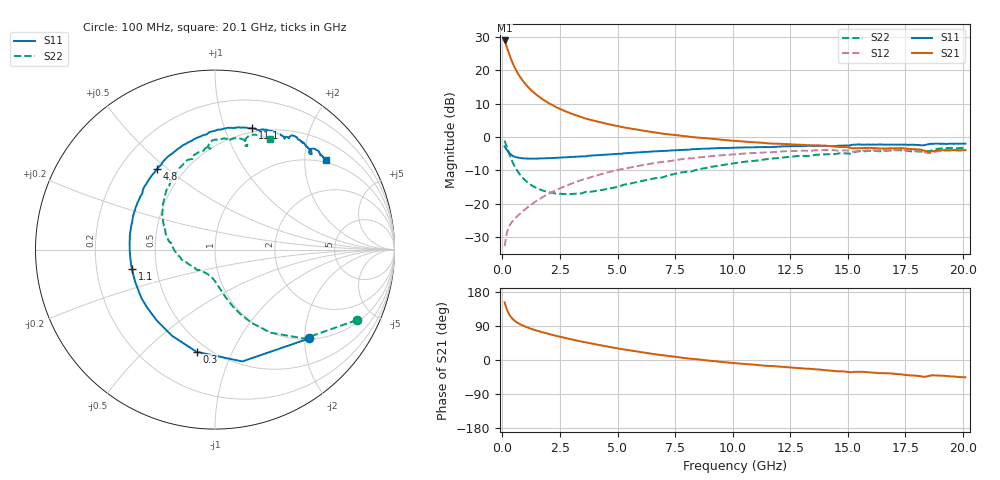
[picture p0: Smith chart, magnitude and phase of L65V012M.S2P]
!  Infineon Technologies AG
! BFR380L3 , PF131585-7, No.6, Th 09.10.01, soldered on pcb-board, measured with PP GSG850
!  Vce=5.0 V,  Ic=12.5 mA
! Common Emitter S-Parameters:  15. November 2001
#  GHz  S  MA  R  50
! f  S11  S21  S12  S22
! GHz  Mag  Ang  Mag  Ang  Mag  Ang  Mag  Ang
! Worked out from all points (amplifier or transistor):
!   201 points, 100 MHz to 20.1 GHz, reference 50 ohm
!   highest |S21| = 28.9 dB at 100 MHz (marker M1)
!   |S21| within 3 dB of that: start of sweep to 245.7 MHz
!   unconditionally stable (mu >= 1): 1.742 GHz to 4.426 GHz
!   at 3.4 GHz: K = 1.03, MAG = 8.5 dB, |S12| = -13.0 dB
!   at 10.1 GHz: K = 0.94, MSG = 2.0 dB, |S12| = -5.2 dB
!   at 20.1 GHz: K = 0.99, MSG = 0.1 dB, |S12| = -4.0 dB
!   S11 on the Smith chart (normalised r, x): 100 MHz: 1.02, -2.11; 300 MHz: 0.43, -0.74; 1.1 GHz: 0.36, -0.10; 4.8 GHz: 0.35, +0.46; 11.1 GHz: 0.46, +1.25; 20.1 GHz: 0.93, +2.53
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0.1  0.7217 -43.3  27.95 152.2  0.02316 69.7  0.8813 -26.5
0.2  0.6415 -76.3  22.06 132.6  0.03745 58.6  0.7028 -44.8
0.3  0.5788 -100.2  17.38 120.1  0.04633 53.3  0.5573 -56.2
0.4  0.5365 -116.6  14.06 111.5  0.05248 51.0  0.4551 -63.5
0.5  0.5115 -129.3  11.7 105.4  0.05753 51.1  0.3838 -68.7
0.6  0.4978 -138.8  9.978 100.7  0.06279 51.6  0.3327 -72.5
0.7  0.4914 -146.4  8.694 96.8  0.06771 52.6  0.2938 -75.5
0.8  0.4831 -152.5  7.685 93.5  0.07286 53.8  0.2645 -78.1
0.9  0.4795 -157.9  6.884 90.6  0.07798 54.7  0.2414 -80.2
1.1  0.4751 -166.7  5.706 85.7  0.08872 56.4  0.209 -84.3
1.3  0.474 -173.5  4.869 81.4  0.09979 57.6  0.1863 -87.8
1.5  0.4753 -179.5  4.254 77.5  0.1111 58.4  0.1711 -91.3
2  0.4817 168.5  3.245 69.0  0.1403 59.1  0.1495 -100.3
2.6  0.4942 157.1  2.546 60.0  0.1763 58.2  0.1408 -112.0
3.5  0.5113 142.6  1.95 47.9  0.2311 54.9  0.145 -128.6
4.8  0.5539 125.7  1.507 32.8  0.3078 48.3  0.1732 -155.0
6.8  0.6147 104.5  1.148 13.7  0.4179 35.6  0.2454 172.2
10.1  0.6943 79.0  0.8737 -8.2  0.5522 14.1  0.4059 134.0
11.1  0.7074 72.9  0.8282 -13.4  0.5819 7.5  0.4476 124.1
13.5  0.733 61.2  0.7515 -24.1  0.6277 -7.3  0.5334 103.3
16.8  0.7681 48.7  0.6773 -35.2  0.6363 -23.9  0.6285 80.4
20.1  0.7961 38.9  0.6386 -45.7  0.6293 -37.9  0.6873 63.3
